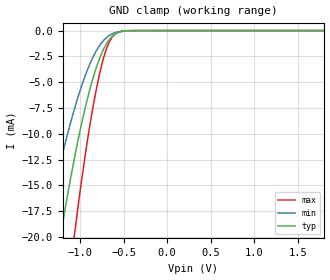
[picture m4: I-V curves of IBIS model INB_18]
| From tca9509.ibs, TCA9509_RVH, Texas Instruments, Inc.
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[Model]   INB_18
Model_type  Input
Vinl=0.15
Vinh=1.26
| variable   typ   min   max
C_comp   1.61pF   1.16pF   1.86pF
[Temperature Range]   40   100   -40
| Ambient temperature   25   85   -40
[Voltage range]   1.8   1.65   1.95
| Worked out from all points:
|   GND clamp passes 1 mA (typ) near -0.68 V on its own axis
[GND Clamp]
| INB_18
|   Voltage   I(typ)   I(min)   I(max)
-1.8V     -55.53mA   -37.93mA   -84.39mA
-1.395V   -29.2mA    -19.21mA   -45.68mA
-1.215V   -19.37mA   -12.38mA   -30.7mA
-1.065V   -12.32mA   -7.569mA   -19.74mA
-1.05V    -11.68mA   -7.139mA   -18.73mA
-930mV    -7.063mA   -4.101mA   -11.39mA
-840mV    -4.263mA   -2.36mA    -6.822mA
-740mV    -1.966mA   -1.047mA   -2.926mA
-660mV    -825.4uA   -449.9uA   -1.019mA
-580mV    -253.7uA   -159uA     -230.8uA
-460mV    -25.6uA    -23.29uA   -12.99uA
1.8V      196.2pA    1.052nA    29.84pA
